(* Logix 5000 AddOnInstructionDefinition export B256_MODL; software revision 30.00 *)

ADD_ON_INSTRUCTION D_SHR   (* revision 1.0, vendor Ken Fischer, NSWCPD, C512 *)
// DINT bit shift right of the 32-bit argument Inp_A by Inp_B bits with paddding by zeros on the right
// Revision note:
// Rev1.0: TBD - Initial Release
VAR_IN_OUT
   Inp_A : DINT; {required}   // 64-bit Integer to be right circular rotated
END_VAR
VAR_INPUT
   Inp_B : INT; {required}   // Number of bits to shift
END_VAR
VAR_IN_OUT
   Out : DINT; {required}   // Result
END_VAR
VAR
   BSR_Cntrl : CONTROL := (LEN := 32);
   ONS : BOOL;
   Source_Bit : BOOL;
   Wrk_InpA : DINT[2];
END_VAR

ROUTINE Logic   (* ladder *)
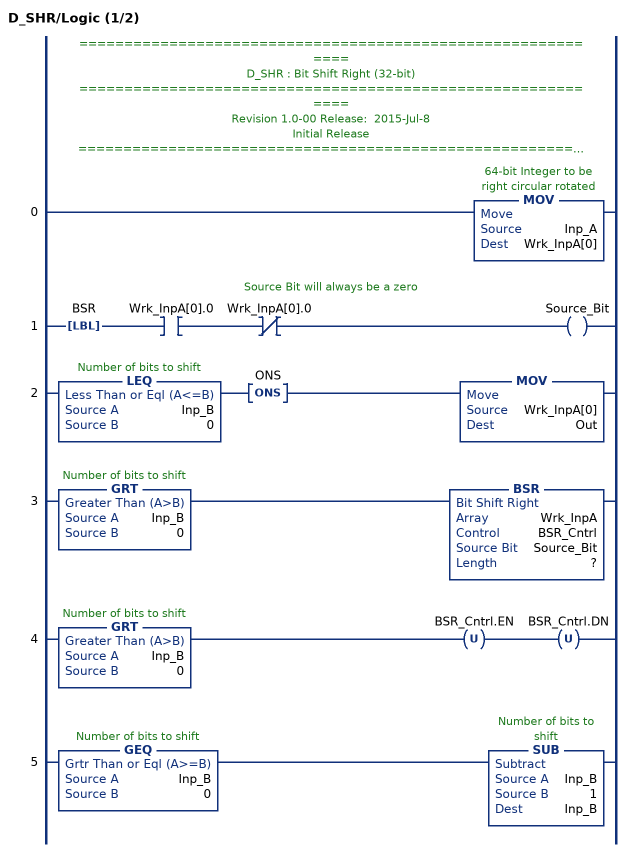
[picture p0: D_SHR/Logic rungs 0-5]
   // ============================================================
   // D_SHR : Bit Shift Right (32-bit)
   // ============================================================
   // Revision 1.0-00 Release:  2015-Jul-8
   // Initial Release
   // ============================================================
   // Performs a right bit shift of the 32-bit argument Inp_A by the
   // number of bits defined in the 16-bit argument Inp_B, with padding by zeros.
   0: MOV(Inp_A,Wrk_InpA[0]);
   // Source Bit will always be a zero
   1: LBL(BSR)XIC(Wrk_InpA[0].0)XIO(Wrk_InpA[0].0)OTE(Source_Bit);
   2: LEQ(Inp_B,0)ONS(ONS)MOV(Wrk_InpA[0],Out);
   3: GRT(Inp_B,0)BSR(Wrk_InpA,BSR_Cntrl,Source_Bit,?);
   4: GRT(Inp_B,0)OTU(BSR_Cntrl.EN)OTU(BSR_Cntrl.DN);
   5: GEQ(Inp_B,0)SUB(Inp_B,1,Inp_B);
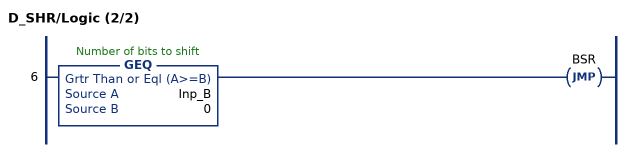
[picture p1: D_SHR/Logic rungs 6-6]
   6: GEQ(Inp_B,0)JMP(BSR);
END_ROUTINE
END_ADD_ON_INSTRUCTION

ADD_ON_INSTRUCTION D_SHL   (* revision 1.0, vendor Ken Fischer, NSWCPD, C512 *)
// DINT bit shift left of the 32-bit argument Inp_A by Inp_B bits with paddding by zeros on the right
// Revision note:
// Rev1.0: TBD - Initial Release
VAR_IN_OUT
   Inp_A : DINT; {required}   // 64-bit Integer to be right circular rotated
END_VAR
VAR_INPUT
   Inp_B : INT; {required}   // Number of bits to shift
END_VAR
VAR_IN_OUT
   Out : DINT; {required}   // Result
END_VAR
VAR
   Wrk_InpA : DINT[2];
   Source_Bit : BOOL;
   ONS : BOOL;
   BSL_Cntrl : CONTROL := (LEN := 32);
END_VAR

ROUTINE Logic   (* ladder *)
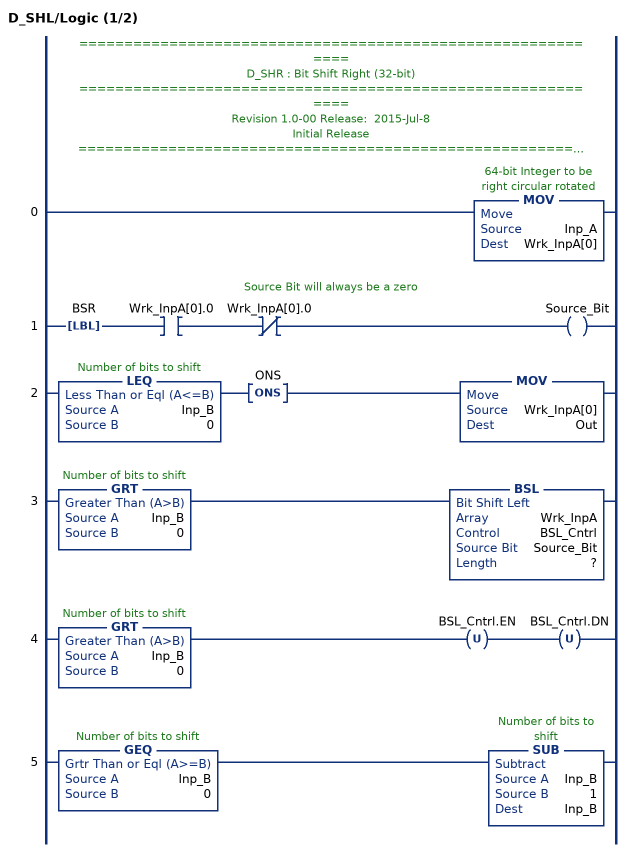
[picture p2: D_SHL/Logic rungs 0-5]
   // ============================================================
   // D_SHR : Bit Shift Right (32-bit)
   // ============================================================
   // Revision 1.0-00 Release:  2015-Jul-8
   // Initial Release
   // ============================================================
   // Performs a left bit shift of the 32-bit argument Inp_A by the
   // number of bits defined in the 16-bit argument Inp_B, with padding by zeros.
   0: MOV(Inp_A,Wrk_InpA[0]);
   // Source Bit will always be a zero
   1: LBL(BSR)XIC(Wrk_InpA[0].0)XIO(Wrk_InpA[0].0)OTE(Source_Bit);
   2: LEQ(Inp_B,0)ONS(ONS)MOV(Wrk_InpA[0],Out);
   3: GRT(Inp_B,0)BSL(Wrk_InpA,BSL_Cntrl,Source_Bit,?);
   4: GRT(Inp_B,0)OTU(BSL_Cntrl.EN)OTU(BSL_Cntrl.DN);
   5: GEQ(Inp_B,0)SUB(Inp_B,1,Inp_B);
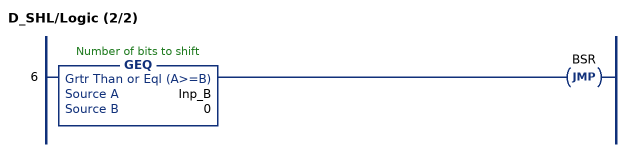
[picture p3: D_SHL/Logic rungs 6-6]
   6: GEQ(Inp_B,0)JMP(BSR);
END_ROUTINE
END_ADD_ON_INSTRUCTION

ADD_ON_INSTRUCTION B256_CtoE   (* revision 1.0 20170916, vendor Kenneth A. Fischer *)
// Convert 256-bit value using 22 12-bit pieces into 256-bit value using 32 8-bit pieces
// Revision note:
// Rev1.0: 20170916 - Initial Release
VAR_IN_OUT
   Inp_C : DINT[22]; {required}
   Out_E : DINT[32]; {required}
END_VAR
VAR
   i : INT;
   j : INT;
   TEMP1 : DINT;
   TEMP2 : DINT;
   D_SHL : D_SHL;
   D_SHR : D_SHR;
END_VAR

ROUTINE Logic   (* ladder *)
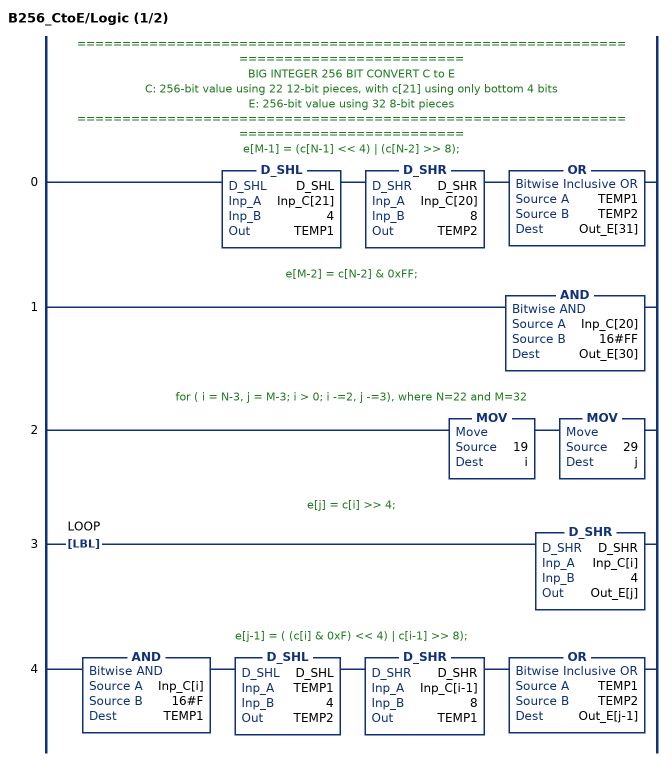
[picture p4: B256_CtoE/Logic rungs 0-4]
   // ======================================================================================
   // BIG INTEGER 256 BIT CONVERT C to E
   // C: 256-bit value using 22 12-bit pieces, with c[21] using only bottom 4 bits
   // E: 256-bit value using 32 8-bit pieces
   // ======================================================================================
   // e[M-1] = (c[N-1] << 4) | (c[N-2] >> 8);
   0: D_SHL(D_SHL,Inp_C[21],4,TEMP1)D_SHR(D_SHR,Inp_C[20],8,TEMP2)OR(TEMP1,TEMP2,Out_E[31]);
   // e[M-2] = c[N-2] & 0xFF;
   1: AND(Inp_C[20],16#FF,Out_E[30]);
   // for ( i = N-3, j = M-3; i > 0; i -=2, j -=3), where N=22 and M=32
   2: MOV(19,i)MOV(29,j);
   // e[j] = c[i] >> 4;
   3: LBL(LOOP)D_SHR(D_SHR,Inp_C[i],4,Out_E[j]);
   // e[j-1] = ( (c[i] & 0xF) << 4) | c[i-1] >> 8);
   4: AND(Inp_C[i],16#F,TEMP1)D_SHL(D_SHL,TEMP1,4,TEMP2)D_SHR(D_SHR,Inp_C[i-1],8,TEMP1)OR(TEMP1,TEMP2,Out_E[j-1]);
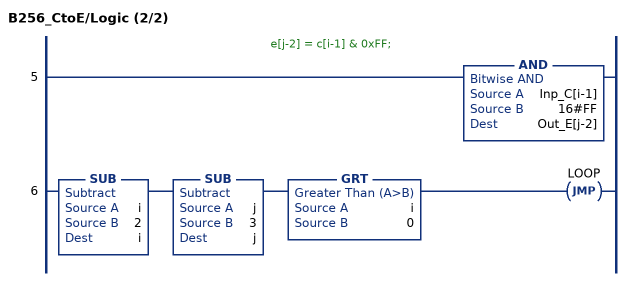
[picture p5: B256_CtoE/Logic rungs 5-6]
   // e[j-2] = c[i-1] & 0xFF;
   5: AND(Inp_C[i-1],16#FF,Out_E[j-2]);
   6: SUB(i,2,i)SUB(j,3,j)GRT(i,0)JMP(LOOP);
END_ROUTINE
END_ADD_ON_INSTRUCTION

ADD_ON_INSTRUCTION B256_MODL   (* revision 1.0 20170916, vendor Kenneth A. Fischer *)
// e = d mod L
// L is curve group order
// Revision note:
// Rev1.0: 20170916 - Initial Release
VAR_IN_OUT
   Temp_C : DINT[22]; {required}
   Temp_D : DINT[43]; {required}
   Inp_D : DINT[43]; {required}   // V
   Out_E : DINT[32]; {required}   // U
END_VAR
VAR_INPUT
   SEQCTRL_RESET : BOOL;   // Resets Mod_L if Toggled True
END_VAR
VAR_OUTPUT
   SEQCTRL_DN : BOOL; {access Read Only}   // Complete
   SEQCTRL_STEP : INT; {access Read Only}
   i : INT; {access Read Only}
END_VAR
VAR
   SEQCTRL_CMD : INT;
   SEQCTRL_DONE : INT;
   SEQCTRL_NEXT_STEP : INT;
   j : INT;
   SEQCTRL_CMD_TABLE : INT[100];
   k : INT;
   p : INT;
   t : DINT;
   carry : DINT;
   s : DINT;
   q : INT;
   TEMP : INT;
   L : DINT[22];
   TEMPDINT : DINT;
   D_SHR : D_SHR;
   negative : DINT;
   B256_CtoE : B256_CtoE;
END_VAR

ROUTINE Logic   (* ladder *)
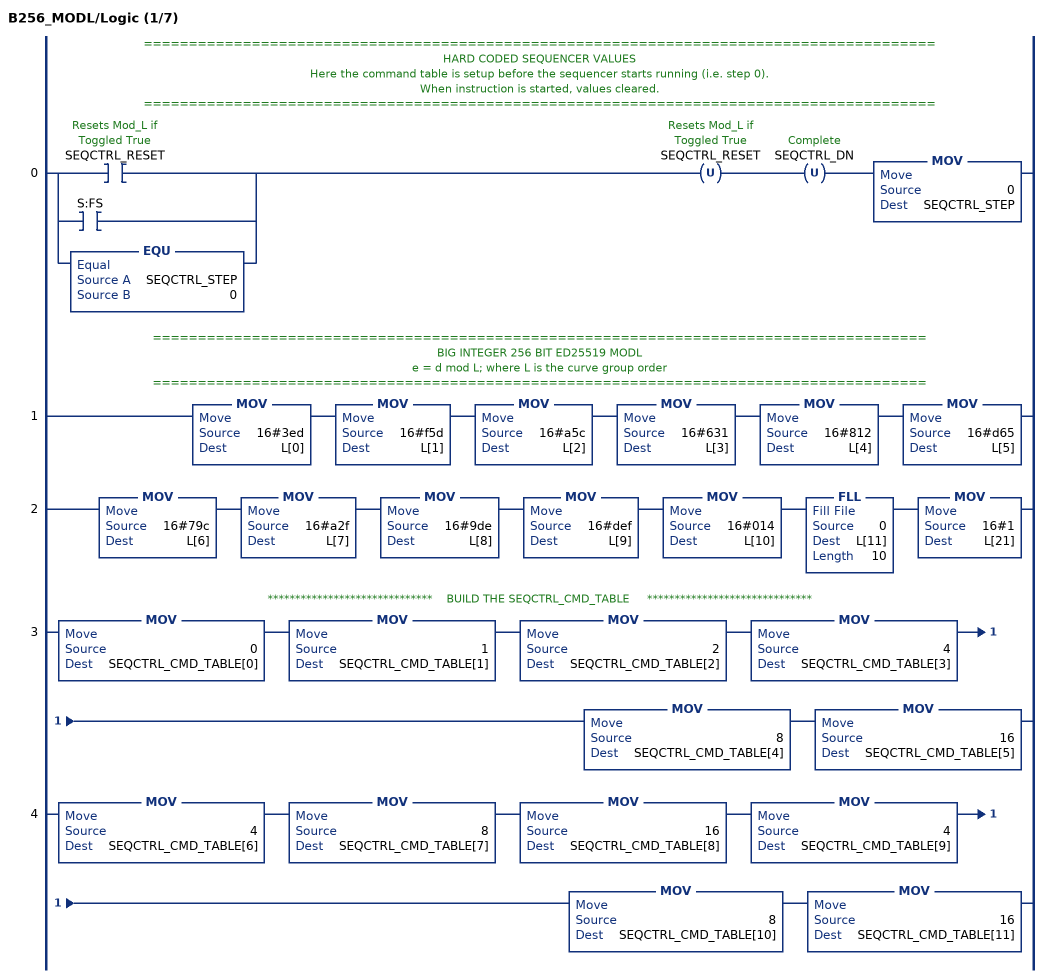
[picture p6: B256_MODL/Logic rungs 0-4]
   // ========================================================================================
   // HARD CODED SEQUENCER VALUES
   // Here the command table is setup before the sequencer starts running (i.e. step 0).
   // When instruction is started, values cleared.
   // ========================================================================================
   0: [[XIC(SEQCTRL_RESET) ,XIC(S:FS) ] ,EQU(SEQCTRL_STEP,0) ]OTU(SEQCTRL_RESET)OTU(SEQCTRL_DN)MOV(0,SEQCTRL_STEP);
   // ======================================================================================
   // BIG INTEGER 256 BIT ED25519 MODL
   //  e = d mod L; where L is the curve group order
   // ======================================================================================
   1: MOV(16#3ed,L[0])MOV(16#f5d,L[1])MOV(16#a5c,L[2])MOV(16#631,L[3])MOV(16#812,L[4])MOV(16#d65,L[5]);
   2: MOV(16#79c,L[6])MOV(16#a2f,L[7])MOV(16#9de,L[8])MOV(16#def,L[9])MOV(16#014,L[10])FLL(0,L[11],10)MOV(16#1,L[21]);
   // ******************************    BUILD THE SEQCTRL_CMD_TABLE     ******************************
   3: MOV(0,SEQCTRL_CMD_TABLE[0])MOV(1,SEQCTRL_CMD_TABLE[1])MOV(2,SEQCTRL_CMD_TABLE[2])MOV(4,SEQCTRL_CMD_TABLE[3])MOV(8,SEQCTRL_CMD_TABLE[4])MOV(16,SEQCTRL_CMD_TABLE[5]);
   4: MOV(4,SEQCTRL_CMD_TABLE[6])MOV(8,SEQCTRL_CMD_TABLE[7])MOV(16,SEQCTRL_CMD_TABLE[8])MOV(4,SEQCTRL_CMD_TABLE[9])MOV(8,SEQCTRL_CMD_TABLE[10])MOV(16,SEQCTRL_CMD_TABLE[11]);
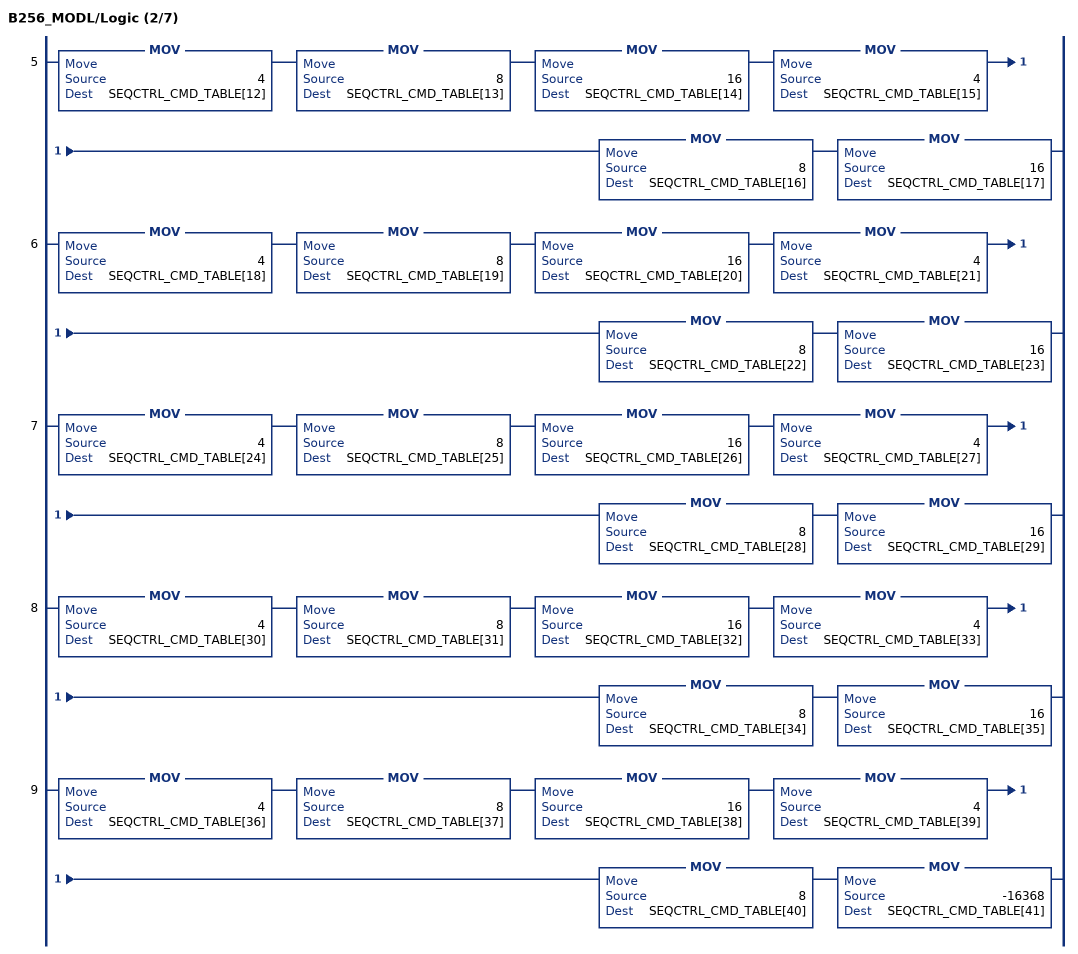
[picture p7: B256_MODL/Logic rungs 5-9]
   5: MOV(4,SEQCTRL_CMD_TABLE[12])MOV(8,SEQCTRL_CMD_TABLE[13])MOV(16,SEQCTRL_CMD_TABLE[14])MOV(4,SEQCTRL_CMD_TABLE[15])MOV(8,SEQCTRL_CMD_TABLE[16])MOV(16,SEQCTRL_CMD_TABLE[17]);
   6: MOV(4,SEQCTRL_CMD_TABLE[18])MOV(8,SEQCTRL_CMD_TABLE[19])MOV(16,SEQCTRL_CMD_TABLE[20])MOV(4,SEQCTRL_CMD_TABLE[21])MOV(8,SEQCTRL_CMD_TABLE[22])MOV(16,SEQCTRL_CMD_TABLE[23]);
   7: MOV(4,SEQCTRL_CMD_TABLE[24])MOV(8,SEQCTRL_CMD_TABLE[25])MOV(16,SEQCTRL_CMD_TABLE[26])MOV(4,SEQCTRL_CMD_TABLE[27])MOV(8,SEQCTRL_CMD_TABLE[28])MOV(16,SEQCTRL_CMD_TABLE[29]);
   8: MOV(4,SEQCTRL_CMD_TABLE[30])MOV(8,SEQCTRL_CMD_TABLE[31])MOV(16,SEQCTRL_CMD_TABLE[32])MOV(4,SEQCTRL_CMD_TABLE[33])MOV(8,SEQCTRL_CMD_TABLE[34])MOV(16,SEQCTRL_CMD_TABLE[35]);
   9: MOV(4,SEQCTRL_CMD_TABLE[36])MOV(8,SEQCTRL_CMD_TABLE[37])MOV(16,SEQCTRL_CMD_TABLE[38])MOV(4,SEQCTRL_CMD_TABLE[39])MOV(8,SEQCTRL_CMD_TABLE[40])MOV(-16368,SEQCTRL_CMD_TABLE[41]);
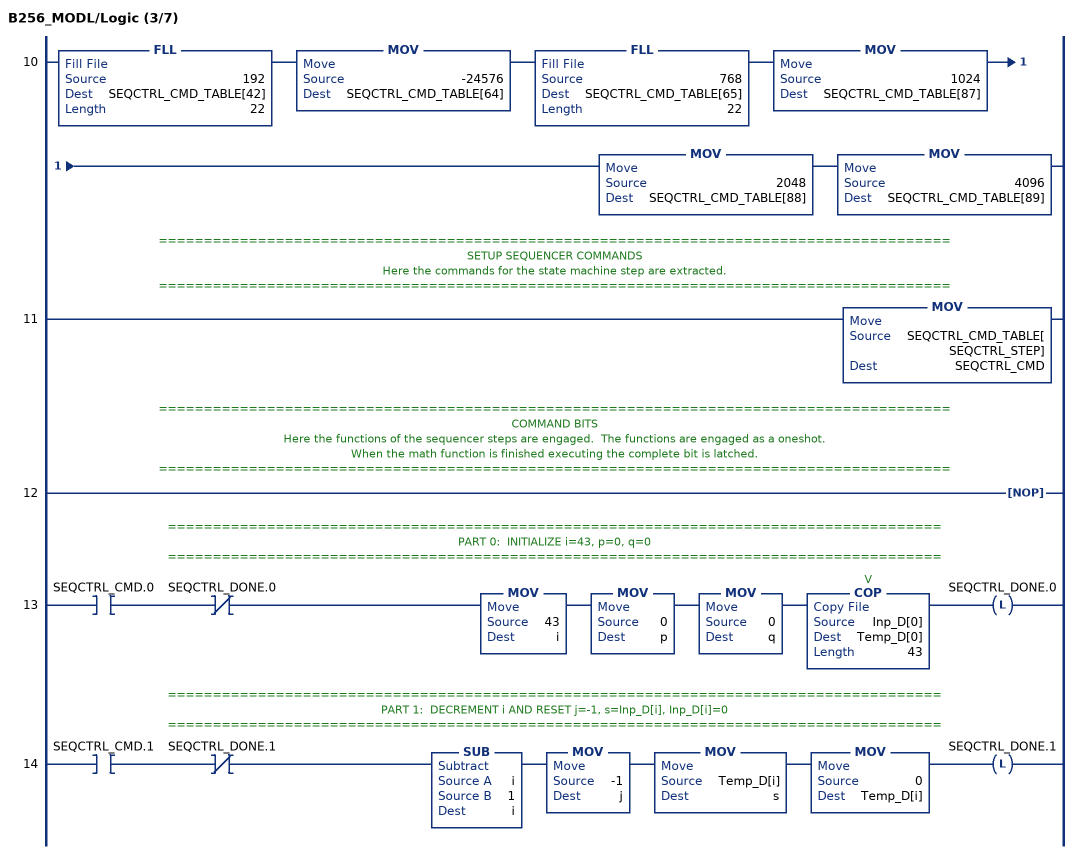
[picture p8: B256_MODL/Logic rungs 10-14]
   10: FLL(192,SEQCTRL_CMD_TABLE[42],22)MOV(-24576,SEQCTRL_CMD_TABLE[64])FLL(768,SEQCTRL_CMD_TABLE[65],22)MOV(1024,SEQCTRL_CMD_TABLE[87])MOV(2048,SEQCTRL_CMD_TABLE[88])MOV(4096,SEQCTRL_CMD_TABLE[89]);
   // ========================================================================================
   // SETUP SEQUENCER COMMANDS
   // Here the commands for the state machine step are extracted.
   // ========================================================================================
   11: MOV(SEQCTRL_CMD_TABLE[SEQCTRL_STEP],SEQCTRL_CMD);
   // ========================================================================================
   // COMMAND BITS
   // Here the functions of the sequencer steps are engaged.  The functions are engaged as a oneshot.
   // When the math function is finished executing the complete bit is latched.
   // ========================================================================================
   12: NOP();
   // ======================================================================================
   // PART 0:  INITIALIZE i=43, p=0, q=0
   // ======================================================================================
   13: XIC(SEQCTRL_CMD.0)XIO(SEQCTRL_DONE.0)MOV(43,i)MOV(0,p)MOV(0,q)COP(Inp_D[0],Temp_D[0],43)OTL(SEQCTRL_DONE.0);
   // ======================================================================================
   // PART 1:  DECREMENT i AND RESET j=-1, s=Inp_D[i], Inp_D[i]=0
   // ======================================================================================
   14: XIC(SEQCTRL_CMD.1)XIO(SEQCTRL_DONE.1)SUB(i,1,i)MOV(-1,j)MOV(Temp_D[i],s)MOV(0,Temp_D[i])OTL(SEQCTRL_DONE.1);
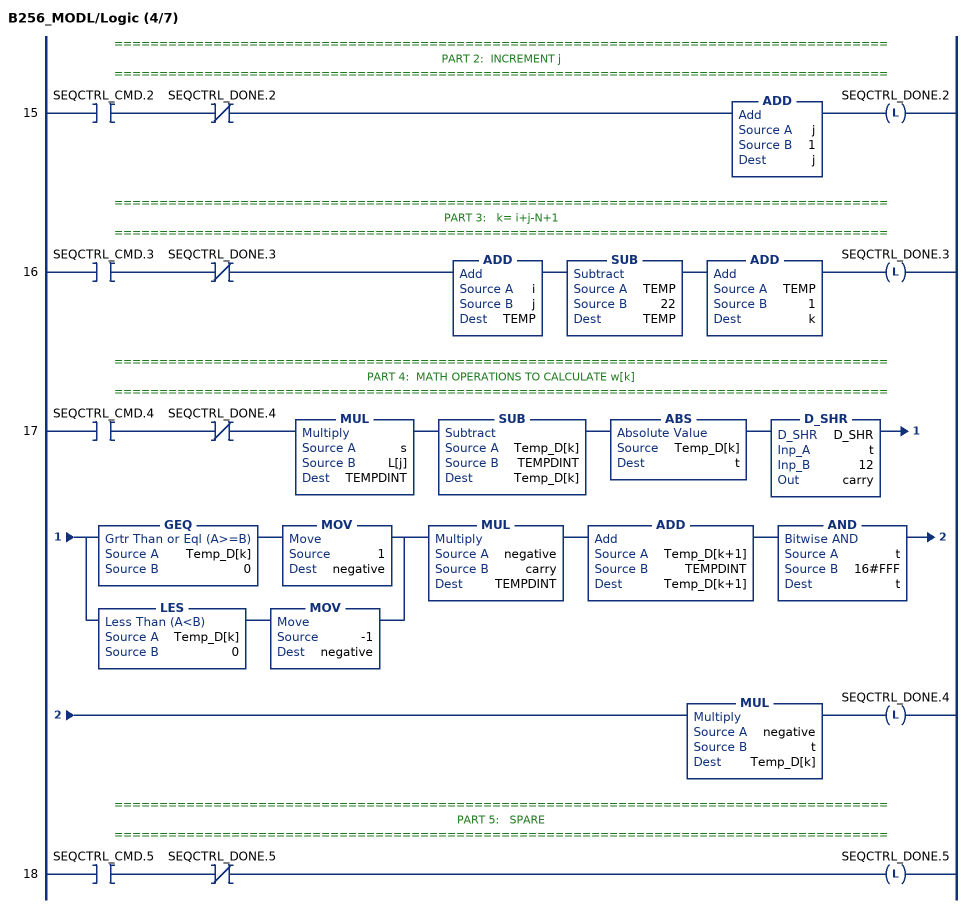
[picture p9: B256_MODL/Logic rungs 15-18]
   // ======================================================================================
   // PART 2:  INCREMENT j
   // ======================================================================================
   15: XIC(SEQCTRL_CMD.2)XIO(SEQCTRL_DONE.2)ADD(j,1,j)OTL(SEQCTRL_DONE.2);
   // ======================================================================================
   // PART 3:   k= i+j-N+1
   // ======================================================================================
   16: XIC(SEQCTRL_CMD.3)XIO(SEQCTRL_DONE.3)ADD(i,j,TEMP)SUB(TEMP,22,TEMP)ADD(TEMP,1,k)OTL(SEQCTRL_DONE.3);
   // ======================================================================================
   // PART 4:  MATH OPERATIONS TO CALCULATE w[k]
   // ======================================================================================
   17: XIC(SEQCTRL_CMD.4)XIO(SEQCTRL_DONE.4)MUL(s,L[j],TEMPDINT)SUB(Temp_D[k],TEMPDINT,Temp_D[k])ABS(Temp_D[k],t)D_SHR(D_SHR,t,12,carry)[GEQ(Temp_D[k],0) MOV(1,negative) ,LES(Temp_D[k],0) MOV(-1,negative) ]MUL(negative,carry,TEMPDINT)ADD(Temp_D[k+1],TEMPDINT,Temp_D[k+1])AND(t,16#FFF,t)MUL(negative,t,Temp_D[k])OTL(SEQCTRL_DONE.4);
   // ======================================================================================
   // PART 5:   SPARE
   // ======================================================================================
   18: XIC(SEQCTRL_CMD.5)XIO(SEQCTRL_DONE.5)OTL(SEQCTRL_DONE.5);
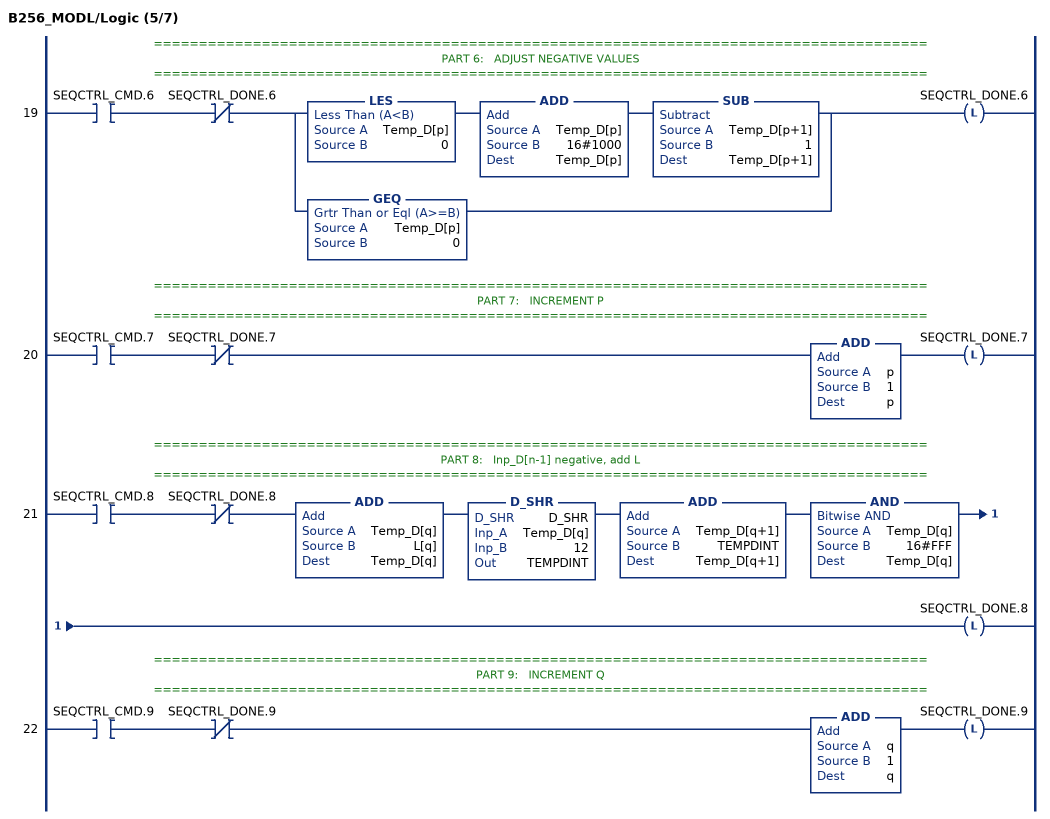
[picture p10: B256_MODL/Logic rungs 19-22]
   // ======================================================================================
   // PART 6:   ADJUST NEGATIVE VALUES
   // ======================================================================================
   19: XIC(SEQCTRL_CMD.6)XIO(SEQCTRL_DONE.6)[LES(Temp_D[p],0) ADD(Temp_D[p],16#1000,Temp_D[p]) SUB(Temp_D[p+1],1,Temp_D[p+1]) ,GEQ(Temp_D[p],0) ]OTL(SEQCTRL_DONE.6);
   // ======================================================================================
   // PART 7:   INCREMENT P
   // ======================================================================================
   20: XIC(SEQCTRL_CMD.7)XIO(SEQCTRL_DONE.7)ADD(p,1,p)OTL(SEQCTRL_DONE.7);
   // ======================================================================================
   // PART 8:   Inp_D[n-1] negative, add L
   // ======================================================================================
   21: XIC(SEQCTRL_CMD.8)XIO(SEQCTRL_DONE.8)ADD(Temp_D[q],L[q],Temp_D[q])D_SHR(D_SHR,Temp_D[q],12,TEMPDINT)ADD(Temp_D[q+1],TEMPDINT,Temp_D[q+1])AND(Temp_D[q],16#FFF,Temp_D[q])OTL(SEQCTRL_DONE.8);
   // ======================================================================================
   // PART 9:   INCREMENT Q
   // ======================================================================================
   22: XIC(SEQCTRL_CMD.9)XIO(SEQCTRL_DONE.9)ADD(q,1,q)OTL(SEQCTRL_DONE.9);
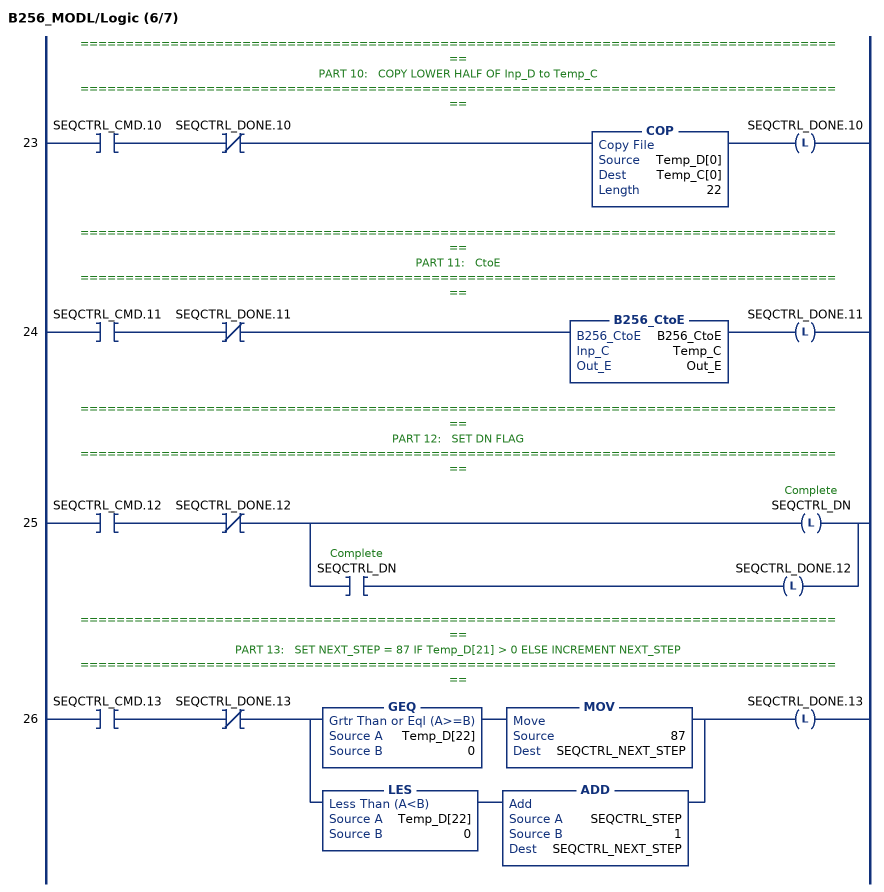
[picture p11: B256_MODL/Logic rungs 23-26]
   // ======================================================================================
   // PART 10:   COPY LOWER HALF OF Inp_D to Temp_C
   // ======================================================================================
   23: XIC(SEQCTRL_CMD.10)XIO(SEQCTRL_DONE.10)COP(Temp_D[0],Temp_C[0],22)OTL(SEQCTRL_DONE.10);
   // ======================================================================================
   // PART 11:   CtoE
   // ======================================================================================
   24: XIC(SEQCTRL_CMD.11)XIO(SEQCTRL_DONE.11)B256_CtoE(B256_CtoE,Temp_C,Out_E)OTL(SEQCTRL_DONE.11);
   // ======================================================================================
   // PART 12:   SET DN FLAG
   // ======================================================================================
   25: XIC(SEQCTRL_CMD.12)XIO(SEQCTRL_DONE.12)[OTL(SEQCTRL_DN) ,XIC(SEQCTRL_DN) OTL(SEQCTRL_DONE.12) ];
   // ======================================================================================
   // PART 13:   SET NEXT_STEP = 87 IF Temp_D[21] > 0 ELSE INCREMENT NEXT_STEP
   // ======================================================================================
   26: XIC(SEQCTRL_CMD.13)XIO(SEQCTRL_DONE.13)[GEQ(Temp_D[22],0) MOV(87,SEQCTRL_NEXT_STEP) ,LES(Temp_D[22],0) ADD(SEQCTRL_STEP,1,SEQCTRL_NEXT_STEP) ]OTL(SEQCTRL_DONE.13);
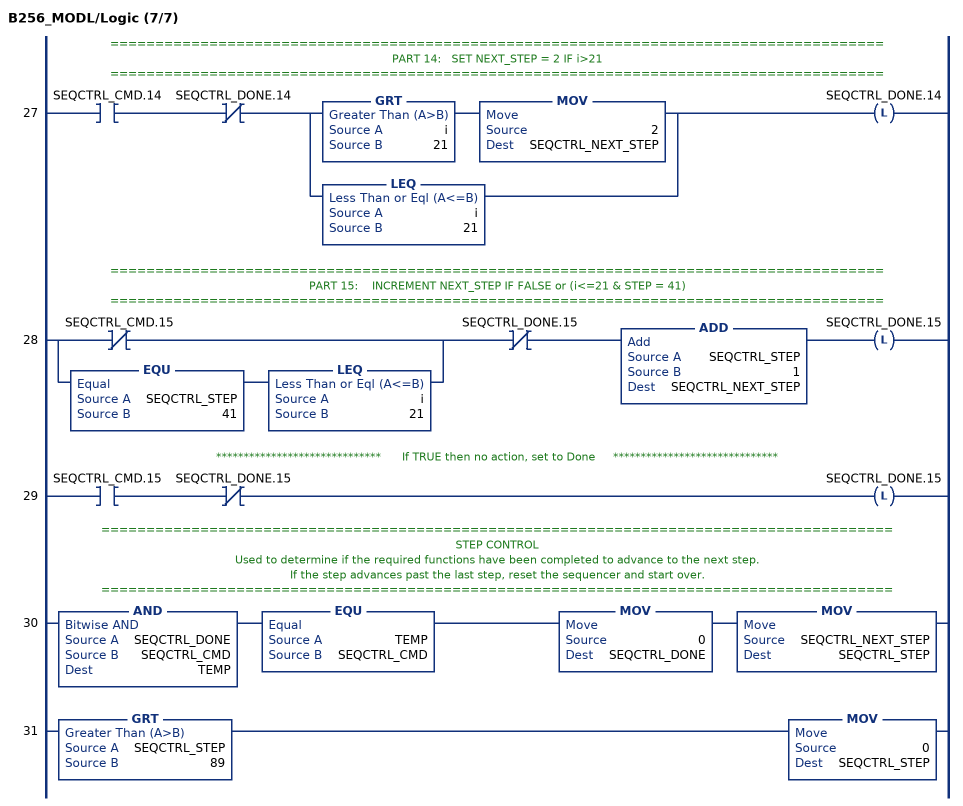
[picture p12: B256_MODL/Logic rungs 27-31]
   // ======================================================================================
   // PART 14:   SET NEXT_STEP = 2 IF i>21
   // ======================================================================================
   27: XIC(SEQCTRL_CMD.14)XIO(SEQCTRL_DONE.14)[GRT(i,21) MOV(2,SEQCTRL_NEXT_STEP) ,LEQ(i,21) ]OTL(SEQCTRL_DONE.14);
   // ======================================================================================
   // PART 15:    INCREMENT NEXT_STEP IF FALSE or (i<=21 & STEP = 41)
   // ======================================================================================
   28: [XIO(SEQCTRL_CMD.15) ,EQU(SEQCTRL_STEP,41) LEQ(i,21) ]XIO(SEQCTRL_DONE.15)ADD(SEQCTRL_STEP,1,SEQCTRL_NEXT_STEP)OTL(SEQCTRL_DONE.15);
   // ******************************      If TRUE then no action, set to Done     ******************************
   29: XIC(SEQCTRL_CMD.15)XIO(SEQCTRL_DONE.15)OTL(SEQCTRL_DONE.15);
   // ========================================================================================
   // STEP CONTROL
   // Used to determine if the required functions have been completed to advance to the next step.
   // If the step advances past the last step, reset the sequencer and start over.
   // ========================================================================================
   30: AND(SEQCTRL_DONE,SEQCTRL_CMD,TEMP)EQU(TEMP,SEQCTRL_CMD)MOV(0,SEQCTRL_DONE)MOV(SEQCTRL_NEXT_STEP,SEQCTRL_STEP);
   31: GRT(SEQCTRL_STEP,89)MOV(0,SEQCTRL_STEP);
END_ROUTINE
END_ADD_ON_INSTRUCTION
